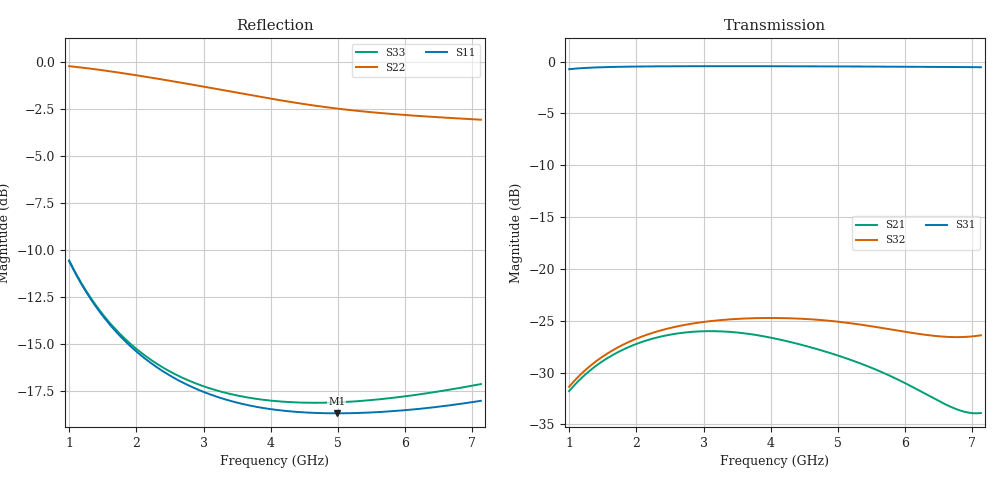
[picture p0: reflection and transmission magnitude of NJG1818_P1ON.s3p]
! Created Mon Jul  5 11:58:54 2021
# hz S ma R 50
! 3 Port Network Data from SP1.SP block
! freq  magS11  angS11  magS12  angS12  magS13  angS13
!  magS21  angS21
!  magS22  angS22  magS23  angS23
!  magS31  angS31  magS32  angS32
!  magS33  angS33
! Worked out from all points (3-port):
!   1226 points, 1 GHz to 7.125 GHz, reference 50 ohm
!   strongest paths, dB at 1 GHz, 2.53 GHz, 4.065 GHz, 5.595 GHz, 7.125 GHz:
!     S31: -0.7, -0.5, -0.5, -0.5, -0.5
!     S32: -31.4, -25.7, -24.7, -25.6, -26.4
!     S21: -31.8, -26.3, -26.7, -29.8, -33.9
!   lowest |S11| = -18.7 dB at 4.98 GHz (marker M1), VSWR 1.26, Z = 46.3 - j10.6 ohm
!   |S11| at or under -10 dB: start of sweep to end of sweep
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1e9  0.2956 -73.2  0.0257 66.7  0.9183 10.8
     0.0257 66.7  0.9726 -36.1  0.02699 70.8
     0.9183 10.8  0.02699 70.8  0.2967 -73.1
1.665e9  0.1948 -80.3  0.03867 52.5  0.942 0.5
         0.03867 52.5  0.9395 -58.6  0.04076 59.5
         0.942 0.5  0.04076 59.5  0.197 -79.9
2.335e9  0.1532 -84.7  0.04689 39.6  0.9479 -6.3
         0.04689 39.6  0.8998 -79.6  0.05017 50.0
         0.9479 -6.3  0.05017 50.0  0.1565 -83.9
2.755e9  0.1388 -87.3  0.04943 32.4  0.9492 -9.8
         0.04943 32.4  0.8737 -91.8  0.05391 45.2
         0.9492 -9.8  0.05391 45.2  0.143 -86.0
3.225e9  0.1285 -90.2  0.04998 25.2  0.9497 -13.4
         0.04998 25.2  0.8443 -104.6  0.05648 40.9
         0.9497 -13.4  0.05648 40.9  0.1336 -88.4
4.065e9  0.1191 -95.9  0.04609 15.9  0.949 -19.4
         0.04609 15.9  0.7939 -125.0  0.05792 35.6
         0.949 -19.4  0.05792 35.6  0.1256 -92.7
4.98e9  0.1165 -103.0  0.03836 12.4  0.9471 -25.5
        0.03836 12.4  0.7508 -144.2  0.05569 33.1
        0.9471 -25.5  0.05569 33.1  0.1246 -97.7
6.03e9  0.1189 -112.2  0.02775 18.5  0.9438 -32.4
        0.02775 18.5  0.721 -163.7  0.04951 37.8
        0.9438 -32.4  0.04951 37.8  0.1295 -104.1
6.745e9  0.1229 -118.8  0.02114 37.7  0.9408 -37.1
         0.02114 37.7  0.7074 -176.4  0.04685 48.9
         0.9408 -37.1  0.04685 48.9  0.1355 -108.8
7.125e9  0.1258 -122.4  0.02016 56.8  0.9389 -39.6
         0.02016 56.8  0.7011 177.0  0.0478 57.1
         0.9389 -39.6  0.0478 57.1  0.1393 -111.5
